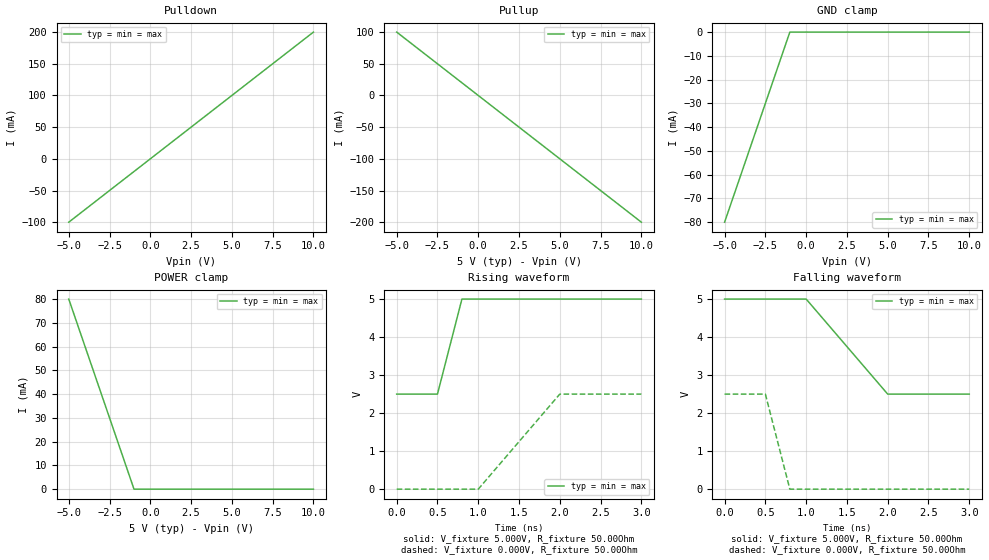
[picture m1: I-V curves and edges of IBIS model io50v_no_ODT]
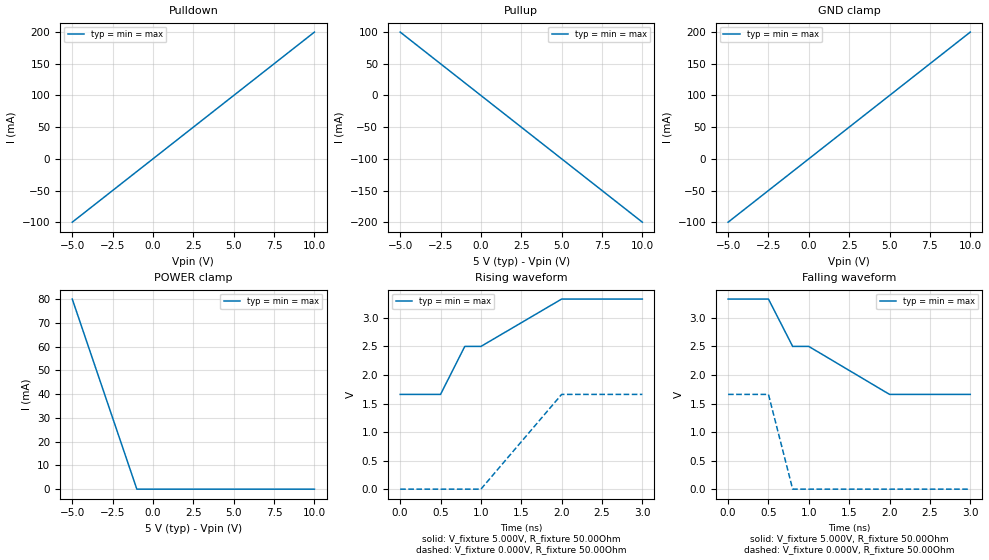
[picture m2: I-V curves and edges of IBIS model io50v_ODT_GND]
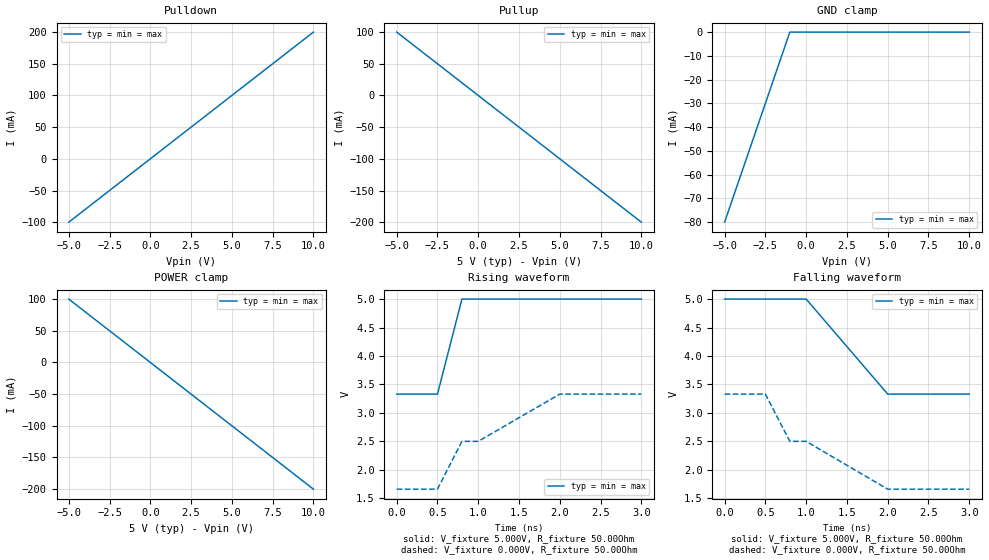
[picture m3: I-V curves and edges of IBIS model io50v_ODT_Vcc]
[IBIS Ver]   3.2
[File Name]   test_ams.ibs
[File Rev]   0.00
[Date]   9/28/2005
[Source]   From silicon level SPICE model at Noname Corporation.
[Notes]   The following information corresponds to the noname chip.
[Disclaimer]   This information is for teaching purposes only and is not
   guaranteed.
[Copyright]   Copyright 2005, Noname Corporation, All Rights Reserved.
[Component]   Test_AMS
[Manufacturer]  Noname Corporation
[Package]
|   typ   min   max
R_pkg   0.0   0.0   0.0
L_pkg   0.0nH   0.0nH   0.0nH
C_pkg   0.0pF   0.0pF   0.0pF
[PIN]   signal_name   model_name   R_pin   L_pin   C_pin
1   Vcc   Power
2   GND   GND
3   IO5_full   io50v_full
4   IO5_no_ODT   io50v_no_ODT
5   IO5_ODT_GND   io50v_ODT_GND
6   IO5_ODT_Vcc   io50v_ODT_Vcc
7   IO5_ODT_Vcc_GND io50v_ODT_Vcc_GND
8   IO5_OSink   io50v_OSink
9   IO5_OSrc   io50v_OSrc
| Models and submodels in the file (7): io50v_no_ODT (I/O), io50v_ODT_GND (I/O), io50v_ODT_Vcc (I/O), io50v_ODT_Vcc_GND (I/O), io50v_OSink (I/O_open_sink), io50v_OSrc (I/O_open_source), io50v_full (I/O)
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[Model]   io50v_no_ODT
Model_type   I/O
Vinl = 800.000mV
Vinh = 2.000V
Vmeas = 1.400V
Vref = 1.400V
Cref = 0.000F
Rref = 50.000Ohm
|   typ   min   max
C_comp   5.000pF   5.000pF   5.000pF
[Voltage Range]   5.000V   5.000V   5.000V
[Temperature Range]   50.0   100.0   0.0
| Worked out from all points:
|   slope of the pulldown table from 0 to 0.75 V, typ, clamps not added: 50 ohm
|   slope of the pullup table from 0 to 0.75 V, typ, clamps not added: 50 ohm
|   falling waveform, V_fixture 5.000V, R_fixture 50.00Ohm: 20-80 % time 600ps typ, 600ps min, 600ps max; typ from 5 V to 2.5 V
|   falling waveform, V_fixture 0.000V, R_fixture 50.00Ohm: 20-80 % time 180ps typ, 180ps min, 180ps max; typ from 2.5 V to 0 V
|   rising waveform, V_fixture 5.000V, R_fixture 50.00Ohm: 20-80 % time 180ps typ, 180ps min, 180ps max; typ from 2.5 V to 5 V
|   rising waveform, V_fixture 0.000V, R_fixture 50.00Ohm: 20-80 % time 600ps typ, 600ps min, 600ps max; typ from 0 V to 2.5 V
[Pulldown]
|   Voltage   I(typ)   I(min)   I(max)
-5V       -100mA     -100mA     -100mA
0V        0A         0A         0A
5V        100mA      100mA      100mA
10V       200mA      200mA      200mA
[GND Clamp]
|   Voltage   I(typ)   I(min)   I(max)
-5V       -80mA      -80mA      -80mA
-1V       0A         0A         0A
5V        0A         0A         0A
10V       0A         0A         0A
[Pullup]
|   Voltage   I(typ)   I(min)   I(max)
-5V       100mA      100mA      100mA
0V        0A         0A         0A
5V        -100mA     -100mA     -100mA
10V       -200mA     -200mA     -200mA
[POWER Clamp]
|   Voltage   I(typ)   I(min)   I(max)
-5V       80mA       80mA       80mA
-1V       0A         0A         0A
5V        0A         0A         0A
10V       0A         0A         0A
[Ramp]
R_load = 50.00Ohm
|   typ   min   max
dV/dt_r   1.403V/1.248ns   1.116V/1.589ns   1.750V/927.496ps
dV/dt_f   1.513V/1.385ns   1.201V/1.726ns   1.878V/1.020ns
[Falling Waveform]
V_fixture = 5.000V
V_fixture_min = 5.000V
V_fixture_max = 5.000V
R_fixture = 50.00Ohm
|   Time   V(typ)   V(min)   V(max)
0s        5V         5V         5V
1ns       5V         5V         5V
2ns       2.5V       2.5V       2.5V
3ns       2.5V       2.5V       2.5V
[Falling Waveform]
V_fixture = 0.000V
V_fixture_min = 0.000V
V_fixture_max = 0.000V
R_fixture = 50.00Ohm
|   Time   V(typ)   V(min)   V(max)
0s        2.5V       2.5V       2.5V
500ps     2.5V       2.5V       2.5V
800ps     0V         0V         0V
3ns       0V         0V         0V
[Rising Waveform]
V_fixture = 5.000V
V_fixture_min = 5.000V
V_fixture_max = 5.000V
R_fixture = 50.00Ohm
|   Time   V(typ)   V(min)   V(max)
0s        2.5V       2.5V       2.5V
500ps     2.5V       2.5V       2.5V
800ps     5V         5V         5V
3ns       5V         5V         5V
[Rising Waveform]
V_fixture = 0.000V
V_fixture_min = 0.000V
V_fixture_max = 0.000V
R_fixture = 50.00Ohm
|   Time   V(typ)   V(min)   V(max)
0s        0V         0V         0V
1ns       0V         0V         0V
2ns       2.5V       2.5V       2.5V
3ns       2.5V       2.5V       2.5V
[Model]   io50v_ODT_GND
Model_type   I/O
Vinl = 800.000mV
Vinh = 2.000V
Vmeas = 1.400V
Vref = 1.400V
Cref = 0.000F
Rref = 50.000Ohm
|   typ   min   max
C_comp   5.000pF   5.000pF   5.000pF
[Voltage Range]   5.000V   5.000V   5.000V
[Temperature Range]   50.0   100.0   0.0
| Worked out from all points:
|   slope of the pulldown table from 0 to 0.75 V, typ, clamps not added: 50 ohm
|   slope of the pullup table from 0 to 0.75 V, typ, clamps not added: 50 ohm
|   falling waveform, V_fixture 5.000V, R_fixture 50.00Ohm: 20-80 % time 982ps typ, 982ps min, 982ps max; typ from 3.33 V to 1.66 V
|   falling waveform, V_fixture 0.000V, R_fixture 50.00Ohm: 20-80 % time 180ps typ, 180ps min, 180ps max; typ from 1.66 V to 0 V
|   rising waveform, V_fixture 5.000V, R_fixture 50.00Ohm: 20-80 % time 978ps typ, 978ps min, 978ps max; typ from 1.66 V to 3.33 V
|   rising waveform, V_fixture 0.000V, R_fixture 50.00Ohm: 20-80 % time 600ps typ, 600ps min, 600ps max; typ from 0 V to 1.66 V
[Pulldown]
|   Voltage   I(typ)   I(min)   I(max)
-5V       -100mA     -100mA     -100mA
0V        0A         0A         0A
5V        100mA      100mA      100mA
10V       200mA      200mA      200mA
[GND Clamp]
|   Voltage   I(typ)   I(min)   I(max)
-5V       -100mA     -100mA     -100mA
0V        0A         0A         0A
5V        100mA      100mA      100mA
10V       200mA      200mA      200mA
[Pullup]
|   Voltage   I(typ)   I(min)   I(max)
-5V       100mA      100mA      100mA
0V        0A         0A         0A
5V        -100mA     -100mA     -100mA
10V       -200mA     -200mA     -200mA
[POWER Clamp]
|   Voltage   I(typ)   I(min)   I(max)
-5V       80mA       80mA       80mA
-1V       0A         0A         0A
5V        0A         0A         0A
10V       0A         0A         0A
[Ramp]
R_load = 50.00Ohm
|   typ   min   max
dV/dt_r   1.403V/1.248ns   1.116V/1.589ns   1.750V/927.496ps
dV/dt_f   1.513V/1.385ns   1.201V/1.726ns   1.878V/1.020ns
[Falling Waveform]
V_fixture = 5.000V
V_fixture_min = 5.000V
V_fixture_max = 5.000V
R_fixture = 50.00Ohm
|   Time   V(typ)   V(min)   V(max)
0s        3.33V      3.33V      3.33V
500ps     3.33V      3.33V      3.33V
800ps     2.5V       2.5V       2.5V
1ns       2.5V       2.5V       2.5V
2ns       1.66V      1.66V      1.66V
3ns       1.66V      1.66V      1.66V
[Falling Waveform]
V_fixture = 0.000V
V_fixture_min = 0.000V
V_fixture_max = 0.000V
R_fixture = 50.00Ohm
|   Time   V(typ)   V(min)   V(max)
0s        1.66V      1.66V      1.66V
500ps     1.66V      1.66V      1.66V
800ps     0V         0V         0V
3ns       0V         0V         0V
[Rising Waveform]
V_fixture = 5.000V
V_fixture_min = 5.000V
V_fixture_max = 5.000V
R_fixture = 50.00Ohm
|   Time   V(typ)   V(min)   V(max)
0s        1.66V      1.66V      1.66V
500ps     1.66V      1.66V      1.66V
800ps     2.5V       2.5V       2.5V
1ns       2.5V       2.5V       2.5V
2ns       3.33V      3.33V      3.33V
3ns       3.33V      3.33V      3.33V
[Rising Waveform]
V_fixture = 0.000V
V_fixture_min = 0.000V
V_fixture_max = 0.000V
R_fixture = 50.00Ohm
|   Time   V(typ)   V(min)   V(max)
0s        0V         0V         0V
1ns       0V         0V         0V
2ns       1.66V      1.66V      1.66V
3ns       1.66V      1.66V      1.66V
[Model]   io50v_ODT_Vcc
Model_type   I/O
Vinl = 800.000mV
Vinh = 2.000V
Vmeas = 1.400V
Vref = 1.400V
Cref = 0.000F
Rref = 50.000Ohm
|   typ   min   max
C_comp   5.000pF   5.000pF   5.000pF
[Voltage Range]   5.000V   5.000V   5.000V
[Temperature Range]   50.0   100.0   0.0
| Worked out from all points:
|   slope of the pulldown table from 0 to 0.75 V, typ, clamps not added: 50 ohm
|   slope of the pullup table from 0 to 0.75 V, typ, clamps not added: 50 ohm
|   falling waveform, V_fixture 5.000V, R_fixture 50.00Ohm: 20-80 % time 600ps typ, 600ps min, 600ps max; typ from 5 V to 3.33 V
|   falling waveform, V_fixture 0.000V, R_fixture 50.00Ohm: 20-80 % time 982ps typ, 982ps min, 982ps max; typ from 3.33 V to 1.66 V
|   rising waveform, V_fixture 5.000V, R_fixture 50.00Ohm: 20-80 % time 180ps typ, 180ps min, 180ps max; typ from 3.33 V to 5 V
|   rising waveform, V_fixture 0.000V, R_fixture 50.00Ohm: 20-80 % time 978ps typ, 978ps min, 978ps max; typ from 1.66 V to 3.33 V
[Pulldown]
|   Voltage   I(typ)   I(min)   I(max)
-5V       -100mA     -100mA     -100mA
0V        0A         0A         0A
5V        100mA      100mA      100mA
10V       200mA      200mA      200mA
[GND Clamp]
|   Voltage   I(typ)   I(min)   I(max)
-5V       -80mA      -80mA      -80mA
-1V       0A         0A         0A
5V        0A         0A         0A
10V       0A         0A         0A
[Pullup]
|   Voltage   I(typ)   I(min)   I(max)
-5V       100mA      100mA      100mA
0V        0A         0A         0A
5V        -100mA     -100mA     -100mA
10V       -200mA     -200mA     -200mA
[POWER Clamp]
|   Voltage   I(typ)   I(min)   I(max)
-5V       100mA      100mA      100mA
0V        0A         0A         0A
5V        -100mA     -100mA     -100mA
10V       -200mA     -200mA     -200mA
[Ramp]
R_load = 50.00Ohm
|   typ   min   max
dV/dt_r   1.403V/1.248ns   1.116V/1.589ns   1.750V/927.496ps
dV/dt_f   1.513V/1.385ns   1.201V/1.726ns   1.878V/1.020ns
[Falling Waveform]
V_fixture = 5.000V
V_fixture_min = 5.000V
V_fixture_max = 5.000V
R_fixture = 50.00Ohm
|   Time   V(typ)   V(min)   V(max)
0s        5V         5V         5V
1ns       5V         5V         5V
2ns       3.33V      3.33V      3.33V
3ns       3.33V      3.33V      3.33V
[Falling Waveform]
V_fixture = 0.000V
V_fixture_min = 0.000V
V_fixture_max = 0.000V
R_fixture = 50.00Ohm
|   Time   V(typ)   V(min)   V(max)
0s        3.33V      3.33V      3.33V
500ps     3.33V      3.33V      3.33V
800ps     2.5V       2.5V       2.5V
1ns       2.5V       2.5V       2.5V
2ns       1.66V      1.66V      1.66V
3ns       1.66V      1.66V      1.66V
[Rising Waveform]
V_fixture = 5.000V
V_fixture_min = 5.000V
V_fixture_max = 5.000V
R_fixture = 50.00Ohm
|   Time   V(typ)   V(min)   V(max)
0s        3.33V      3.33V      3.33V
500ps     3.33V      3.33V      3.33V
800ps     5V         5V         5V
3ns       5V         5V         5V
[Rising Waveform]
V_fixture = 0.000V
V_fixture_min = 0.000V
V_fixture_max = 0.000V
R_fixture = 50.00Ohm
|   Time   V(typ)   V(min)   V(max)
0s        1.66V      1.66V      1.66V
500ps     1.66V      1.66V      1.66V
800ps     2.5V       2.5V       2.5V
1ns       2.5V       2.5V       2.5V
2ns       3.33V      3.33V      3.33V
3ns       3.33V      3.33V      3.33V
